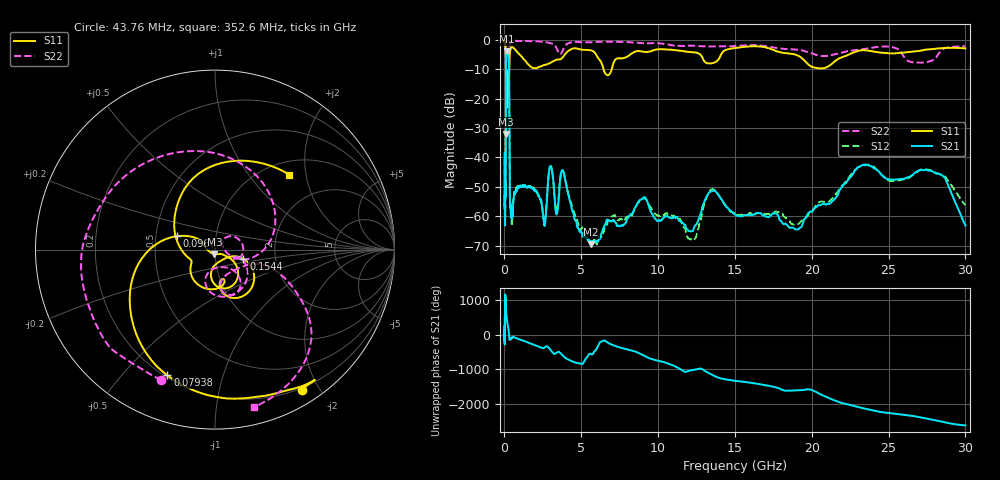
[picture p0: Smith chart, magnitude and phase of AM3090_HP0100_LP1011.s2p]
! Date/Time: Thu, Feb 28, 2019 1:57 PM
! Network Analyzer: Agilent Technologies E8364B Rev: A.07.50.67
! Sweep from 0.010 to 30.000 GHz, 1601 Points, Sweep Type: LOG
! Power Supply: 5.023 V, 0.002 A
# Hz S DB R 50
!freq MagS11 AngS11 MagS21 AngS21 MagS12 AngS12 MagS22 AngS22
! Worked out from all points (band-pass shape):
!   1601 points, 10 MHz to 30 GHz, reference 50 ohm
!   highest |S21| = -3.81 dB at 157.6 MHz (marker M1); lowest = -69.5 dB at 5.64 GHz (marker M2)
!   |S21| within 3 dB of the highest: 106.4 MHz to 284.6 MHz (178.3 MHz wide, 91.2 % of centre)
!   lowest |S11| = -32.0 dB at 104 MHz (marker M3), VSWR 1.05, Z = 49.6 - j2.48 ohm
!   |S11| at or under -10 dB: 94.44 MHz to 314.3 MHz (219.9 MHz wide, 108 % of centre); 6.455 GHz to 6.978 GHz (523.6 MHz wide, 7.8 % of centre)
!   |S22| runs from -27.1 to -0.2 dB; largest |S21 - S12| = 0.015
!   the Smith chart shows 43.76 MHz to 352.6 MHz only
!   S11 on the Smith chart (normalised r, x): 43.76 MHz: 0.18, -1.78; 79.38 MHz: 0.21, -0.67; 96 MHz: 0.64, +0.10; 154.4 MHz: 1.37, -0.14; 352.6 MHz: 1.26, +1.61
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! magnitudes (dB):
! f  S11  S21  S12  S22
! 10 MHz  -0.3  -38.4  -40.5  -0.7
! 38.04 MHz  -0.5  -61.5  -58.6  -1.7
! 43.76 MHz  -0.7  -58.9  -57.4  -2.1
! 79.38 MHz  -2.5  -47.8  -48.2  -4.7
! 96 MHz  -13.0  -14.9  -14.8  -12.6
! 104 MHz  -32.0  -7.6  -7.6  -26.7
! 119.1 MHz  -13.2  -5.1  -5.0  -17.3
! 144.7 MHz  -22.7  -3.9  -3.9  -18.7
! 154.4 MHz  -15.6  -3.8  -3.8  -16.5
! 157.6 MHz  -14.0  -3.8  -3.8  -15.5
! 288.7 MHz  -15.9  -7.4  -7.3  -15.5
! 352.6 MHz  -4.6  -53.5  -52.9  -0.9
! 550.5 MHz  -2.6  -57.8  -55.5  -0.3
! 2.084 GHz  -9.6  -51.7  -51.7  -0.5
! 2.61 GHz  -8.6  -63.3  -61.4  -0.7
! 2.972 GHz  -7.8  -43.1  -43.0  -1.0
! 3.798 GHz  -5.9  -44.5  -44.5  -3.5
! 5.64 GHz  -3.5  -69.5  -70.2  -0.8
! 7.926 GHz  -5.8  -62.1  -60.5  -0.7
! 18.84 GHz  -4.8  -64.1  -62.9  -3.2
! 23.59 GHz  -3.6  -42.6  -42.4  -2.9
! 30 GHz  -2.8  -63.2  -56.3  -2.2
